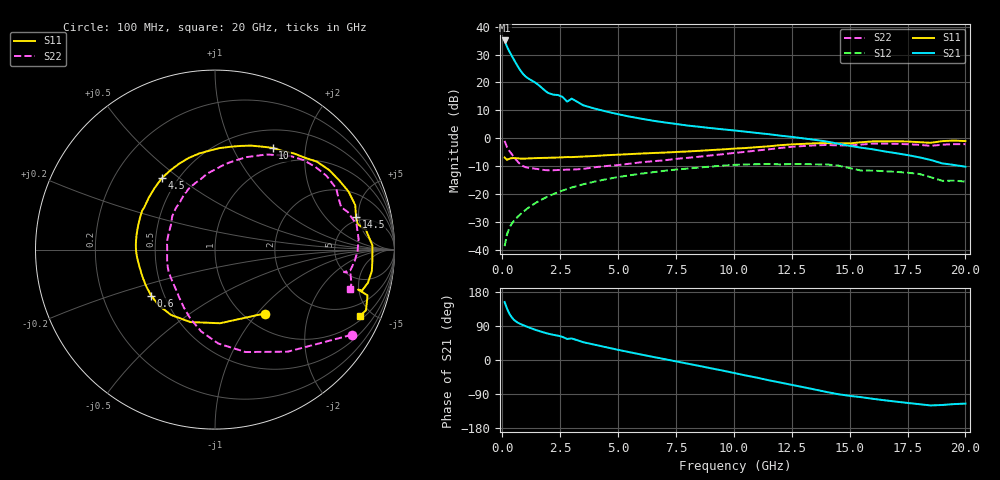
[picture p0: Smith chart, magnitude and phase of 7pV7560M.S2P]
! Infineon Technologies  Discrete & RF Semiconductors
! bfp620
! VCE = 0.75 V,  IC =  60 mA
! Common Emitter S-Parameters:  Sep 2002
# GHz  S  MA  R  50
!  f  S11  S21  S12  S22
! GHz  MAG  ANG  MAG  ANG  MAG  ANG  MAG  ANG
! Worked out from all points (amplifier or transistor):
!   59 points, 100 MHz to 20 GHz, reference 50 ohm
!   highest |S21| = 35.1 dB at 100 MHz (marker M1)
!   |S21| within 3 dB of that: start of sweep to 249.5 MHz
!   unconditionally stable (mu >= 1): 1.893 GHz to 2.297 GHz; 3.156 GHz to 10.51 GHz; 16.92 GHz to end of sweep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
!   at 1 GHz: K = 0.90, MSG = 24.0 dB, |S12| = -25.7 dB
!   at 5.5 GHz: K = 1.05, MAG = 9.2 dB, |S12| = -13.3 dB
!   at 20 GHz: K = 1.50, MAG = -1.5 dB, |S12| = -15.5 dB
!   S11 on the Smith chart (normalised r, x): 100 MHz: 1.22, -1.09; 600 MHz: 0.42, -0.27; 4.5 GHz: 0.41, +0.43; 10 GHz: 0.74, +1.45; 14.5 GHz: 4.47, +4.61; 20 GHz: 1.22, -4.28
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0.1  0.4506 -52.2  56.63 152.8  0.0116 73.5  0.8982 -31.9
0.2  0.4113 -86.1  44.13 136.3  0.0187 62.5  0.6985 -54.5
0.3  0.4264 -108.8  36.35 123.0  0.0243 59.1  0.5954 -73.4
0.4  0.4388 -123.9  30.57 113.2  0.0289 57.8  0.5237 -88.0
0.5  0.4413 -135.2  25.78 106.2  0.0329 57.4  0.4623 -99.6
0.6  0.4384 -144.3  21.76 101.2  0.0366 57.5  0.4093 -109.5
0.8  0.4317 -157.9  16 94.6  0.0439 57.8  0.3357 -126.0
1  0.4315 -166.9  12.88 89.5  0.0516 58.0  0.3029 -138.5
1.4  0.4392 -178.5  10.07 80.3  0.0675 57.1  0.2852 -155.2
1.8  0.4438 171.0  7.403 72.6  0.0834 54.9  0.2698 -171.6
2.6  0.4548 156.3  5.51 60.9  0.1152 48.5  0.2709 168.5
2.8  0.46 152.0  4.53 55.6  0.1229 46.5  0.2733 161.3
3  0.4588 149.8  5.125 56.9  0.1308 44.6  0.2729 161.2
3.5  0.4696 141.4  3.89 46.9  0.1497 39.5  0.2821 150.4
4.5  0.4959 126.8  3.009 33.5  0.1847 29.1  0.3177 133.4
7  0.5526 93.0  1.922 2.5  0.2604 2.8  0.4019 101.0
10  0.6511 60.5  1.381 -34.1  0.3328 -31.0  0.5445 71.2
10.5  0.667 55.4  1.311 -40.7  0.3398 -37.7  0.5697 66.4
13.5  0.8113 23.5  0.936 -77.9  0.3409 -73.1  0.7449 33.5
14.5  0.8064 12.9  0.799 -90.2  0.3235 -88.3  0.7442 21.8
17  0.882 -7.8  0.54 -109.8  0.2493 -103.9  0.7943 -0.6
20  0.8889 -24.5  0.309 -115.1  0.1672 -114.7  0.783 -16.4
